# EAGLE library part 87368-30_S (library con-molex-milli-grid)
RECEPTACAL
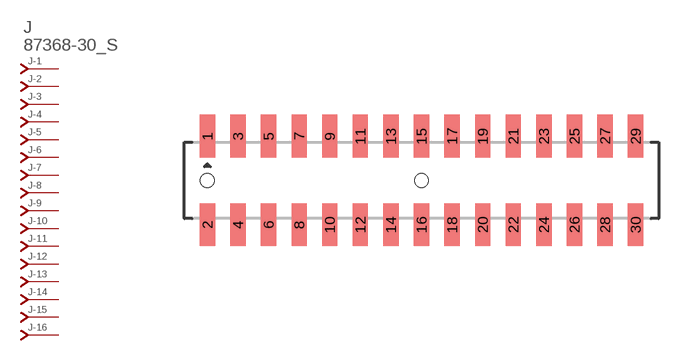
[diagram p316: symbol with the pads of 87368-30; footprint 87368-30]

Designator prefix J; gates -1=J-NV -2=J-N -3=J-N -4=J-N -5=J-N -6=J-N -7=J-N -8=J-N -9=J-N -10=J-N -11=J-N -12=J-N -13=J-N -14=J-N -15=J-N -16=J-N -17=J-N -18=J-N -19=J-N -20=J-N -21=J-N -22=J-N -23=J-N -24=J-N -25=J-N -26=J-N -27=J-N -28=J-N -29=J-N -30=J-N

## 87368-30_S  [87368-30]
1  -1:J  pas
2  -2:J  pas
3  -3:J  pas
4  -4:J  pas
5  -5:J  pas
6  -6:J  pas
7  -7:J  pas
8  -8:J  pas
9  -9:J  pas
10  -10:J  pas
11  -11:J  pas
12  -12:J  pas
13  -13:J  pas
14  -14:J  pas
15  -15:J  pas
16  -16:J  pas
17  -17:J  pas
18  -18:J  pas
19  -19:J  pas
20  -20:J  pas
21  -21:J  pas
22  -22:J  pas
23  -23:J  pas
24  -24:J  pas
25  -25:J  pas
26  -26:J  pas
27  -27:J  pas
28  -28:J  pas
29  -29:J  pas
30  -30:J  pas

## Footprint 87368-30 (pad centres in mm)
RECEPTACAL SMD Dual Row, Side Entry
smd 1 x 2.8: 1 -14,2.9; 2 -14,-2.9; 3 -12,2.9; 4 -12,-2.9; 5 -10,2.9; 6 -10,-2.9; 7 -8,2.9; 8 -8,-2.9; 9 -6,2.9; 10 -6,-2.9; 11 -4,2.9; 12 -4,-2.9; 13 -2,2.9; 14 -2,-2.9; 15 0,2.9; 16 0,-2.9; 17 2,2.9; 18 2,-2.9; 19 4,2.9; 20 4,-2.9; 21 6,2.9; 22 6,-2.9; 23 8,2.9; 24 8,-2.9; 25 10,2.9; 26 10,-2.9; 27 12,2.9; 28 12,-2.9; 29 14,2.9; 30 14,-2.9
hole 0.914 at -14,0
hole 0.914 at 0,0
